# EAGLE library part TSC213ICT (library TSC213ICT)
Current Sense Amplifiers Low / High side bidirectional, zero-drift, current sense amplifiers Source: Datasheet
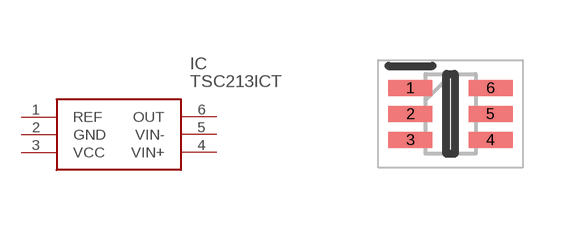
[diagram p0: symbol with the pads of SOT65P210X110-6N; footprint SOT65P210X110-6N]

Designator prefix IC

## TSC213ICT (Arrow_Part_Number: TSC213ICT; Arrow_Price-Stock: https://www.arrow.com/en/products/tsc213ict/stmicroelectronics?region=nac; Description: Current Sense Amplifiers Low / High side bidirectional, zero-drift, current sense amplifiers; Height: 1.1mm; Manufacturer_Name: STMicroelectronics; Manufacturer_Part_Number: TSC213ICT; Mouser_Part_Number: 511-TSC213ICT; Mouser_Price-Stock: https://www.mouser.co.uk/ProductDetail/STMicroelectronics/TSC213ICT?qs=OlC7AqGiEDkXftKCt1OixQ%3D%3D)  [SOT65P210X110-6N]
1  REF
2  GND
3  VCC
4  VIN+
5  VIN-
6  OUT

## Footprint SOT65P210X110-6N (pad centres in mm)
SC70-6_1
smd 1.1 x 0.4: 1 -1,0.65; 2 -1,0; 3 -1,-0.65; 4 1,-0.65; 5 1,0; 6 1,0.65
